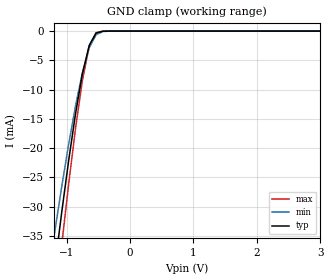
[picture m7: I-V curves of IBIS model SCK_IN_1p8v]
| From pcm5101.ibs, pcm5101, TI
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|   SCK_IN_1p8v
[Model]   SCK_IN_1p8v
Model_type   Input
Vinl = 0.54
Vinh = 1.26
|   typ   min   max
C_comp   1.071750217pF   1.051762612pF   1.095949543pF
[Voltage Range]   1.8   1.65   1.95
[Temperature Range]   27   105   -25
[Power Clamp Reference]   1.8   1.65   1.95
[GND Clamp Reference]   -0   -0   -0
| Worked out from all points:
|   GND clamp passes 1 mA (typ) near -0.57 V on its own axis
[GND Clamp]
|   Voltage   I(typ)   I(min)   I(max)
-1.8V     -98.84mA   -82.48mA   -114.6mA
-1.182V   -40.15mA   -34.09mA   -47.29mA
-1.074V   -30.87mA   -26.51mA   -36.44mA
-966.5mV  -22.14mA   -19.37mA   -26.15mA
-858.5mV  -14.17mA   -12.82mA   -16.66mA
-750.5mV  -7.34mA    -7.15mA    -8.456mA
-642.5mV  -2.44mA    -2.864mA   -2.573mA
-534.5mV  -344.3uA   -626.2uA   -273.2uA
-426.5mV  -20.47uA   -69.77uA   -9.634uA
-318.5mV  -657.5nA   -5.032uA   -138.7nA
3.6V      0A         0A         0A
[POWER Clamp]
|   Voltage   I(typ)   I(min)   I(max)
-1.8V     0A         0A         0A
0V        0A         0A         0A
3.6V      0A         0A         0A
